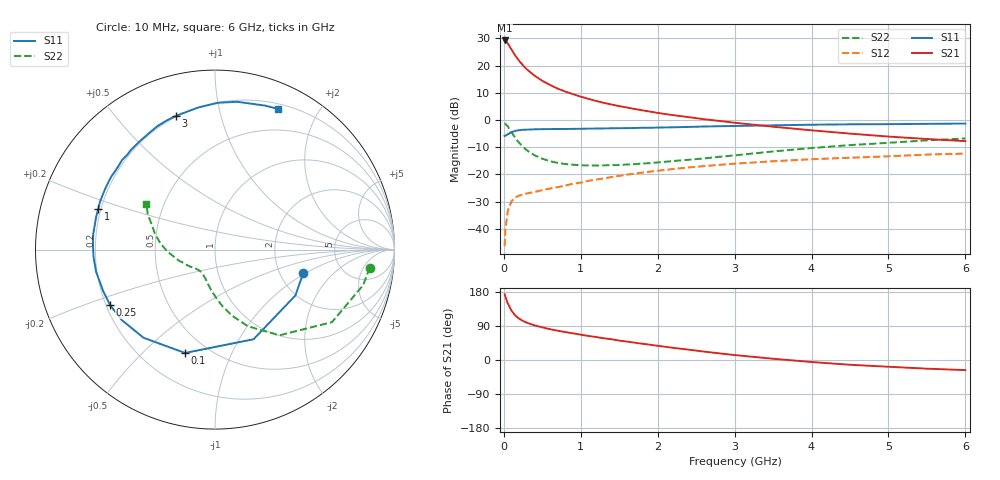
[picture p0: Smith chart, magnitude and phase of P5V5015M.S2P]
! SIEMENS Small Signal Semiconductors
! BFP183
! Si NPN RF Bipolar Junction Transistor in SOT143
! VCE = 0.5 V  IC = 15 mA
! Common Emitter S-Parameters:  March  1996
# GHz  S  MA  R  50
!  f  S11  S21  S12  S22
! GHz  MAG  ANG  MAG  ANG  MAG  ANG  MAG  ANG
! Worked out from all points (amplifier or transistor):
!   36 points, 10 MHz to 6 GHz, reference 50 ohm
!   highest |S21| = 29.2 dB at 10 MHz (marker M1)
!   |S21| within 3 dB of that: start of sweep to 92.57 MHz
!   unconditionally stable (mu >= 1): 499.5 MHz to end of sweep
!   at 250 MHz: K = 0.60, MSG = 23.7 dB, |S12| = -27.4 dB
!   at 1.4 GHz: K = 1.51, MAG = 9.1 dB, |S12| = -21.0 dB
!   at 6 GHz: K = 1.32, MAG = -1.1 dB, |S12| = -12.3 dB
!   S11 on the Smith chart (normalised r, x): 10 MHz: 2.70, -0.94; 100 MHz: 0.38, -0.68; 250 MHz: 0.22, -0.24; 1 GHz: 0.19, +0.16; 3 GHz: 0.19, +0.73; 6 GHz: 0.25, +1.52
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0.01  0.5089 -14.7  28.94 173.7  0.0048 80.3  0.868 -6.7
0.02  0.5158 -29.7  28.66 167.5  0.0096 77.1  0.8487 -13.5
0.05  0.5437 -66.7  25.71 150.1  0.021 64.0  0.7669 -31.8
0.1  0.5996 -106.2  19.69 130.1  0.0322 48.7  0.598 -53.0
0.15  0.6322 -129.0  15.18 117.1  0.0378 40.4  0.4649 -66.8
0.2  0.6511 -142.9  12.19 109.0  0.0408 36.5  0.3786 -75.7
0.25  0.6609 -152.1  10.05 103.0  0.0428 34.8  0.3201 -82.2
0.3  0.6645 -159.6  8.502 98.4  0.0447 34.5  0.2769 -87.6
0.4  0.6739 -169.4  6.508 91.3  0.0476 35.4  0.2242 -95.9
0.5  0.6782 -176.7  5.241 86.1  0.0513 36.1  0.1944 -101.7
0.6  0.6806 177.4  4.411 81.3  0.0549 38.1  0.175 -106.7
0.7  0.6841 172.8  3.77 77.3  0.0584 39.6  0.1626 -111.5
0.8  0.6834 168.7  3.323 73.6  0.0624 40.6  0.155 -115.1
1  0.6887 160.8  2.678 66.8  0.0707 42.4  0.1472 -121.2
1.1  0.6942 157.2  2.445 63.5  0.0762 43.3  0.1462 -124.0
1.5  0.7066 144.6  1.797 51.2  0.0942 43.3  0.1486 -133.9
2.2  0.7343 125.1  1.228 32.2  0.1255 39.3  0.1761 -150.2
3  0.7763 106.3  0.89 13.1  0.1573 32.2  0.2236 -167.8
3.5  0.7975 96.6  0.752 3.3  0.1745 27.7  0.2642 -177.3
4.5  0.8328 81.4  0.562 -12.6  0.2024 18.0  0.3455 165.5
5.5  0.8496 70.7  0.447 -22.9  0.2315 9.7  0.422 152.5
6  0.8594 65.8  0.409 -26.7  0.242 4.9  0.4574 146.6
